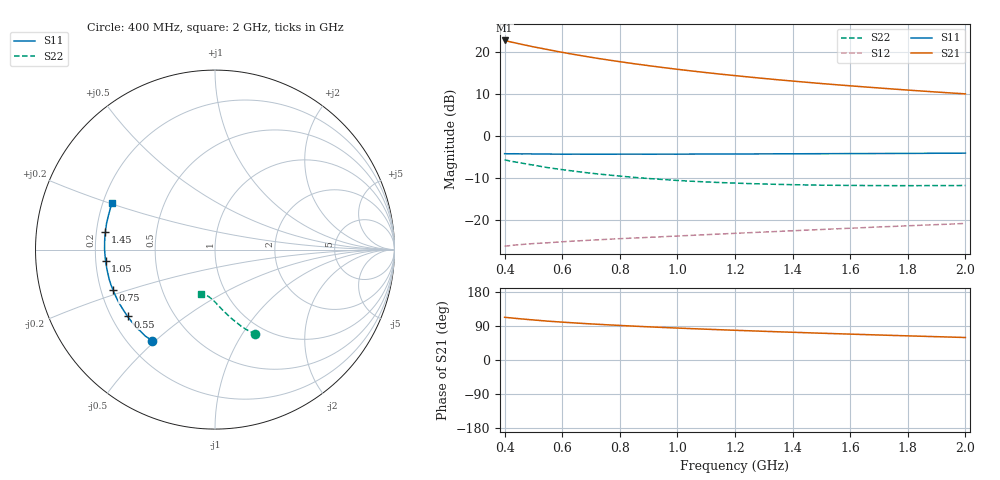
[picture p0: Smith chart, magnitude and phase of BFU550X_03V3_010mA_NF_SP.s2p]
! Filename:  P:\Prog\Test\Noise\ATS_data\Testdata_Net\BFU550X no attenuator noise\BFU550X_APG2013_44_C05_03p3V_010mA_NF_CM01_D.sf
! Date/Time: Fri 26/Jul/2013 14:37:11
! BFU550X_APG2013_44_C05_03p3V_1to10mA_NF_CM01_Bias5_R.sf
! Noise Parameter Data File
! BFU550X_APG2013_44_C05_03p3V_1to10mA_NF_CM01
! Date/time: Wed Jul 24 15:50:55 2013
! VAR V_out= 3.300000
! VAR I_out= 9.995000
! VAR V_in= 0.829800
! VAR I_in= 0.113010
! Device data file deembeded for feedlines and parallel
! Original file: \BFU550X no attenuator noise\BFU550X_APG2013_44_C05_03p3V_010mA_NF_CM01_R.sf
! Feed-files: PR005V01_100713_Feed1.s2p, PR005V01_100713_Feed2.s2p
! Parallel-file: PR005V01_100713_Par.s2p
# MHz S MA R 50
!  Freq-MHz  S11-mag  S11-arg  S21-mag  S21-arg  S12-mag  S12-arg  S22-mag  S22-arg
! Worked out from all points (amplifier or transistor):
!   37 points, 400 MHz to 2 GHz, reference 50 ohm
!   highest |S21| = 22.8 dB at 400 MHz (marker M1)
!   |S21| within 3 dB of that: start of sweep to 614.5 MHz
!   unconditionally stable (mu >= 1): 1.892 GHz to end of sweep
!   at 500 MHz: K = 0.43, MSG = 23.4 dB, |S12| = -25.5 dB
!   at 1.1 GHz: K = 0.78, MSG = 19.3 dB, |S12| = -23.4 dB
!   at 2 GHz: K = 1.01, MAG = 14.7 dB, |S12| = -20.7 dB
!   lowest NFmin = 0.78 dB at 480 MHz
!   S11 on the Smith chart (normalised r, x): 400 MHz: 0.30, -0.49; 550 MHz: 0.27, -0.32; 750 MHz: 0.25, -0.18; 1.05 GHz: 0.24, -0.05; 1.45 GHz: 0.24, +0.07; 2 GHz: 0.24, +0.21
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400  0.6199 -124.3  13.76 112.7  0.04925 42.4  0.5234 -64.5
420  0.6172 -127.0  13.24 111.2  0.05005 41.9  0.5063 -66.0
433  0.6189 -128.8  12.96 110.2  0.05063 41.6  0.4965 -66.8
460  0.6159 -132.2  12.35 108.3  0.05156 40.8  0.4791 -68.6
500  0.6154 -137.1  11.56 105.7  0.05285 39.9  0.4534 -71.0
550  0.6133 -142.6  10.71 102.5  0.05402 39.2  0.4231 -73.6
600  0.6115 -147.1  9.941 99.9  0.05554 38.8  0.4005 -75.9
650  0.612 -151.2  9.269 97.5  0.05681 38.5  0.3805 -78.0
700  0.6112 -154.9  8.678 95.2  0.05804 38.3  0.363 -79.9
750  0.6112 -158.2  8.157 93.2  0.05929 38.3  0.3486 -81.6
800  0.612 -161.4  7.696 91.2  0.06046 38.3  0.3355 -83.4
850  0.6122 -164.3  7.278 89.3  0.06155 38.4  0.3239 -84.9
950  0.6121 -169.6  6.558 85.9  0.06388 38.9  0.3054 -87.7
1050  0.613 -174.2  5.968 82.7  0.06624 39.6  0.2915 -90.1
1100  0.6133 -176.3  5.708 81.2  0.06747 39.8  0.2858 -91.3
1200  0.6153 179.7  5.254 78.4  0.07 40.4  0.2769 -93.5
1300  0.6163 176.1  4.863 75.7  0.07252 41.0  0.2704 -95.5
1450  0.6187 171.0  4.375 71.9  0.07645 41.8  0.2635 -98.3
1500  0.6196 169.4  4.23 70.7  0.07773 42.1  0.2617 -99.2
1600  0.6218 166.3  3.974 68.3  0.08051 42.6  0.26 -100.9
1750  0.6236 162.0  3.637 64.8  0.0846 43.1  0.2583 -103.4
2000  0.6294 155.5  3.188 59.4  0.09183 44.0  0.2596 -107.3
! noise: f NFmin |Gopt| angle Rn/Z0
400  0.816  0.09909  164.9  0.0854
460  0.7819  0.139  174.1  0.0715
600  0.8477  0.1005  163.9  0.087
800  0.8453  0.1886  170.3  0.0656
1000  0.8714  0.2333  171.3  0.0586
1200  0.8998  0.2558  170.7  0.0593
1400  0.9266  0.2824  178.1  0.0574
1600  0.942  0.326  -177.2  0.0518
1800  0.9795  0.3608  -175.3  0.0486
2000  1.01  0.3575  -170.3  0.0573
